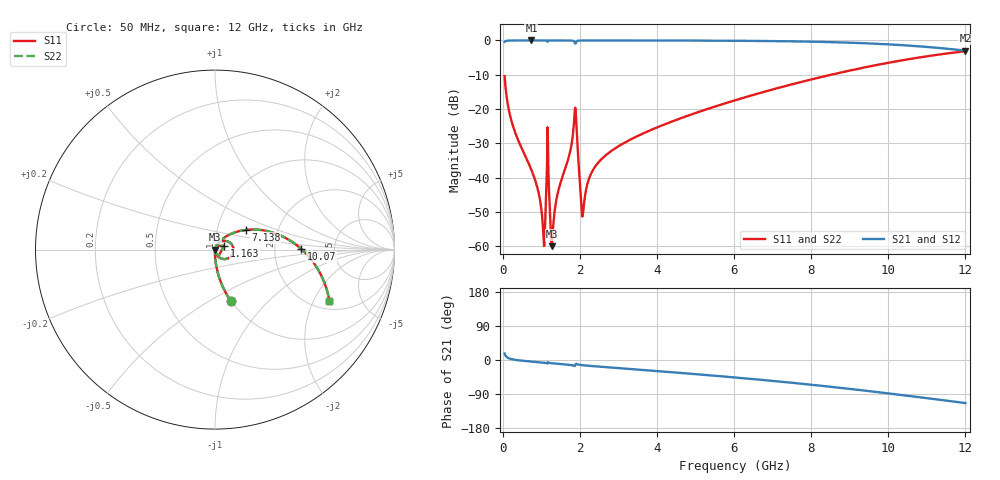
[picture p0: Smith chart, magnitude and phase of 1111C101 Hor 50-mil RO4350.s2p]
# GHz S MA R 50
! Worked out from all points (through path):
!   1601 points, 50 MHz to 12 GHz, reference 50 ohm
!   highest |S21| = -0.01 dB at 744.6 MHz (marker M1); lowest = -3.0 dB at 12 GHz (marker M2)
!   group delay of S21, straight-line fit = 26.2 ps
!   lowest |S11| = -60.0 dB at 1.275 GHz (marker M3), VSWR 1.00, Z = 50.1 + j0.00495 ohm
!   |S11| at or under -10 dB: start of sweep to 8.516 GHz
!   |S22| runs from -60.0 to -3.1 dB; largest |S21 - S12| = 0
!   S11 on the Smith chart (normalised r, x): 50 MHz: 1.00, -0.63; 1.163 GHz: 1.10, +0.05; 7.138 GHz: 1.37, +0.31; 10.07 GHz: 2.84, +0.04; 12 GHz: 2.42, -2.67
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0.05  0.3019 -72.7  0.9531 17.2  0.9531 17.2  0.3019 -72.7
0.2665938  0.05658 -88.1  0.9979 1.5  0.9979 1.5  0.05658 -88.1
0.7445938  0.01299 -91.0  0.9992 -4.2  0.9992 -4.2  0.01299 -91.0
0.9238437  0.006286 -88.4  0.9991 -5.8  0.9991 -5.8  0.006286 -88.4
1.050812  0.001635 -62.0  0.999 -6.9  0.999 -6.9  0.001635 -62.0
1.088156  0.001295 28.3  0.9989 -7.3  0.9989 -7.3  0.001295 28.3
1.162844  0.05418 23.3  0.9539 -9.4  0.9539 -9.4  0.05418 23.3
1.192719  0.008993 -84.6  0.9979 -7.4  0.9979 -7.4  0.008993 -84.6
1.274875  0.001005 2.8  0.9989 -8.5  0.9989 -8.5  0.001005 2.8
1.864906  0.08483 33.2  0.9424 -16.0  0.9424 -16.0  0.08483 33.2
1.924656  0.04174 -65.9  0.9754 -10.8  0.9754 -10.8  0.04174 -65.9
2.044156  0.00347 -40.6  0.9968 -13.4  0.9968 -13.4  0.00347 -40.6
2.096437  0.003573 36.1  0.9976 -14.0  0.9976 -14.0  0.003573 36.1
2.268219  0.01068 66.0  0.9982 -15.6  0.9982 -15.6  0.01068 66.0
2.581906  0.01908 67.7  0.9983 -18.1  0.9983 -18.1  0.01908 67.7
4.038312  0.05503 58.8  0.9966 -29.5  0.9966 -29.5  0.05503 58.8
6.025  0.1342 42.9  0.9884 -46.1  0.9884 -46.1  0.1342 42.9
7.137844  0.2024 32.8  0.9762 -56.5  0.9762 -56.5  0.2024 32.8
8.019156  0.2714 23.9  0.9589 -65.4  0.9589 -65.4  0.2714 23.9
10.01331  0.4735 1.2  0.876 -88.3  0.876 -88.3  0.4735 1.2
10.06559  0.4794 0.6  0.8727 -88.9  0.8727 -88.9  0.4794 0.6
12  0.6971 -24.0  0.7108 -113.6  0.7108 -113.6  0.6971 -24.0
